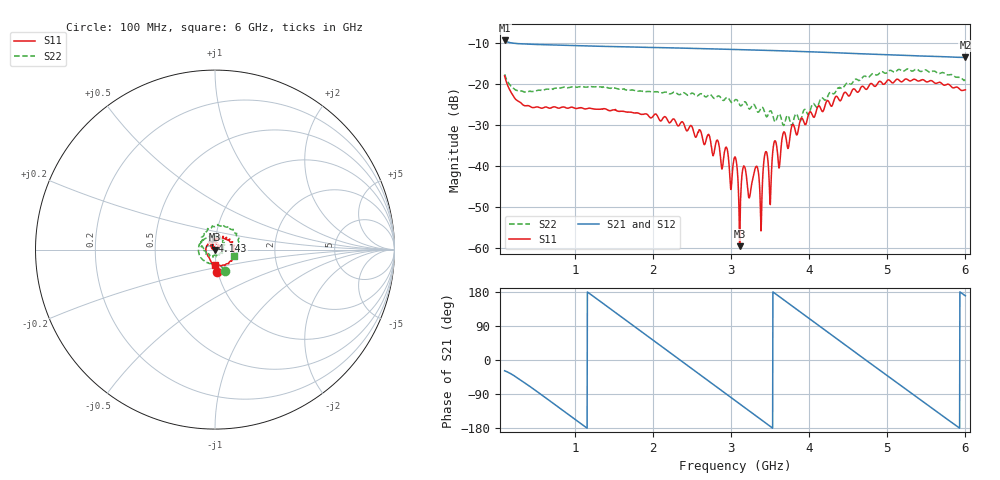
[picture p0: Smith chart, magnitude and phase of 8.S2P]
!Agilent Technologies,E5071C,MY46316741,A.11.02
!Date: Thu Dec 16 09:42:21 2021
!Data & Calibration Information:
!Freq	S11:SOLT4(ON)	S21:SOLT4(ON)	S12:SOLT4(ON)	S22:SOLT4(ON)
!PortZ  Port1:50+j0  Port2:50+j0
!Above PortZ is port z conversion or system Z0 setting when saving the data.
!When reading, reference impedance value at option line is always used.
# Hz S dB R 50
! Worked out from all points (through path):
!   1593 points, 100 MHz to 6 GHz, reference 50 ohm
!   highest |S21| = -9.40 dB at 100 MHz (marker M1); lowest = -13.5 dB at 6 GHz (marker M2)
!   group delay of S21, straight-line fit = 420 ps
!   lowest |S11| = -59.6 dB at 3.109 GHz (marker M3), VSWR 1.00, Z = 50.1 + j0.0164 ohm
!   |S11| at or under -10 dB: start of sweep to end of sweep
!   |S22| runs from -30.2 to -16.4 dB; largest |S21 - S12| = 0.0016
!   S11 on the Smith chart (normalised r, x): 100 MHz: 0.99, -0.25; 4.143 GHz: 0.97, +0.09; 6 GHz: 0.98, -0.17
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1e8  -18.05 -84.7  -9.40 -28.4  -9.41 -28.4  -17.67 -63.8
3.5201e8  -25.31 -129.2  -10.27 -59.4  -10.28 -59.4  -21.97 -90.0
1.085804e9  -25.84 155.3  -10.70 -169.3  -10.70 -169.3  -20.64 -173.2
1.619472e9  -26.70 112.8  -10.95 110.1  -10.95 110.1  -21.26 143.7
2.067902e9  -28.26 85.0  -11.15 42.2  -11.15 42.3  -21.98 116.2
2.823932e9  -33.71 19.1  -11.50 -72.5  -11.51 -72.4  -23.06 58.4
2.998116e9  -45.79 6.8  -11.58 -98.9  -11.59 -98.8  -24.44 47.5
3.05e9  -37.81 7.7  -11.62 -106.7  -11.62 -106.6  -23.94 37.3
3.109296e9  -59.63 9.0  -11.65 -115.8  -11.66 -115.6  -25.11 36.8
3.164887e9  -40.06 10.5  -11.68 -124.1  -11.68 -124.0  -24.46 25.2
3.235302e9  -47.77 -135.4  -11.72 -134.9  -11.72 -134.7  -26.15 19.7
3.327952e9  -40.13 139.2  -11.76 -148.8  -11.77 -148.7  -26.41 11.8
3.379837e9  -53.74 -79.2  -11.79 -156.7  -11.79 -156.5  -26.01 -6.4
3.442839e9  -36.59 140.7  -11.81 -166.3  -11.82 -166.1  -27.70 -9.5
3.49843e9  -49.33 156.2  -11.85 -174.7  -11.85 -174.5  -26.61 -27.3
3.557726e9  -33.95 137.5  -11.88 176.3  -11.88 176.4  -29.15 -34.7
3.617023e9  -40.45 137.3  -11.92 167.3  -11.92 167.5  -27.36 -49.8
3.672613e9  -31.81 134.1  -11.95 158.8  -11.96 159.0  -30.16 -65.6
4.035804e9  -27.42 116.5  -12.19 103.9  -12.19 104.0  -25.19 -156.0
4.143279e9  -25.84 106.6  -12.26 87.6  -12.27 87.7  -23.77 -175.4
5.017902e9  -19.03 12.3  -12.92 -44.1  -12.92 -43.9  -16.88 71.8
6e9  -21.46 -91.4  -13.54 169.3  -13.53 169.6  -19.12 -19.9
